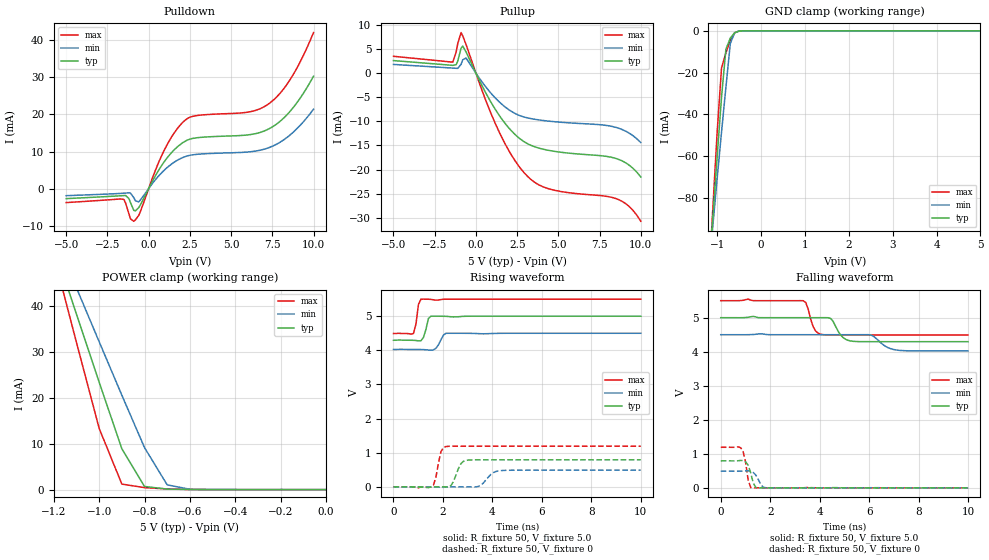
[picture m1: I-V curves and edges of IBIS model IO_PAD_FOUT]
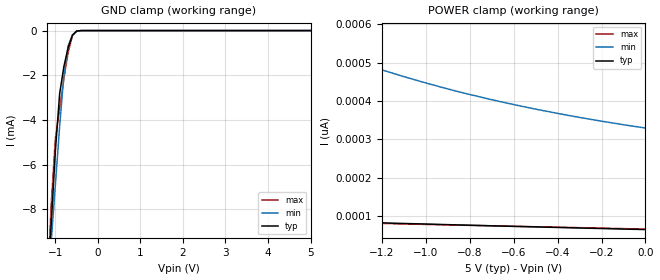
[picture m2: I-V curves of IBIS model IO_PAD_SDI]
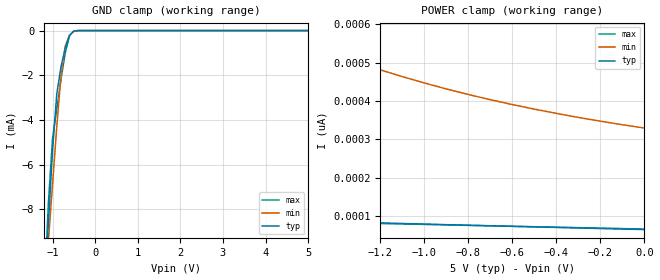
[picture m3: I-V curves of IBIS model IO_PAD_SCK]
[IBIS Ver]   3.2
[Comment Char]   |_char
[File name]   rx4111ce_5v.ibs
[File Rev]   1.0
[Date]   2019/10/04 13:08:42
[Source]
[Notes]
[Disclaimer]
This information is for modeling purposes only, and is not guaranteed.
Property of SEIKO EPSON Corp.,
unauthorized reproduction and/or distribution is strictly prohibited.
[Copyright]
Copyright 2019, SEIKO EPSON Corp.
[Component]   T5462W0A
Si_location Pin
Timing_location Pin
[Manufacturer]   SEIKO EPSON Corp.
| RX-4111CE
[Package]
R_pkg   267m   NA   NA
L_pkg   2.8nH   NA   NA
C_pkg   0.70pF   NA   NA
[Pin] signal_name   model_name
1   VDD   POWER
2   VBAT   POWER
3   DI   IO_PAD_SDI
4   FOUT   IO_PAD_FOUT
5   CLK   IO_PAD_SCK
6   DO   IO_PAD_SDO
7   CE   IO_PAD_CE
8   VIO   POWER
9   GND   GND
10   /INT   IO_PAD_XINT
| Models and submodels in the file (6): IO_PAD_FOUT (3-state), IO_PAD_SDI (Input), IO_PAD_SCK (Input), IO_PAD_SDO (3-state), IO_PAD_CE (Input), IO_PAD_XINT (Open_drain)
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[Model]   IO_PAD_FOUT
Model_type 3-state
Enable Active-High
Polarity Non-Inverting
Vmeas=2.5
C_comp   2.5p   2.0p   3.0p
[Temperature Range] 25   105   -40
[Voltage Range]   5.0   4.5   5.5
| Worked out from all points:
|   slope of the pulldown table from 0 to 0.75 V, typ, clamps not added: 126 ohm
|   slope of the pullup table from 0 to 0.75 V, typ, clamps not added: 149 ohm
|   GND clamp passes 1 mA (typ) near -0.60 V on its own axis
|   POWER clamp passes 1 mA (typ) near -0.80 V on its own axis
|   falling waveform, R_fixture 50, V_fixture 5.0: 20-80 % time 354ps typ, 503ps min, 257ps max; typ from 5 V to 4.29 V
|   falling waveform, R_fixture 50, V_fixture 0: 20-80 % time 185ps typ, 230ps min, 167ps max; typ from 0.793 V to 0 V
|   rising waveform, R_fixture 50, V_fixture 5.0: 20-80 % time 152ps typ, 215ps min, 119ps max; typ from 4.29 V to 5 V
|   rising waveform, R_fixture 50, V_fixture 0: 20-80 % time 269ps typ, 381ps min, 199ps max; typ from 0 V to 0.793 V
[Pullup]
-5V       2.598mA    1.801mA    3.488mA
-1.4V     1.602mA    1.04mA     2.29mA
-1.2V     1.734mA    995.3uA    4.356mA
-900mV    5.147mA    1.814mA    8.407mA
-600mV    4.408mA    3.126mA    5.954mA
1.2V      -7.642mA   -5.236mA   -10.62mA
2.1V      -11.76mA   -7.82mA    -16.67mA
3V        -14.38mA   -9.175mA   -20.93mA
4.5V      -16.07mA   -9.985mA   -24.05mA
8.6V      -17.81mA   -11.36mA   -26.14mA
9.4V      -19.36mA   -12.67mA   -28mA
10V       -21.52mA   -14.39mA   -30.72mA
[Pulldown]
-5V       -2.695mA   -1.899mA   -3.76mA
-1.5V     -1.871mA   -1.232mA   -2.909mA
-1.1V     -3.756mA   -1.223mA   -8.145mA
-900mV    -5.868mA   -2.416mA   -8.805mA
-600mV    -5.116mA   -3.564mA   -7.202mA
900mV     6.952mA    4.772mA    9.936mA
2V        12.16mA    8.239mA    17.55mA
2.7V      13.56mA    9.131mA    19.52mA
6.1V      14.53mA    9.907mA    20.68mA
7.3V      16.12mA    11.06mA    22.91mA
8.6V      20.95mA    14.55mA    29.52mA
10V       30.3mA     21.42mA    42.06mA
[GND Clamp]
-5V       -1.289A    -1.043A    -1.612A
-1.2V     -119.6mA   -117.1mA   -123.7mA
-1.1V     -89.89mA   -93.83mA   -85.8mA
-1V       -60.42mA   -70.86mA   -48.73mA
-900mV    -31.79mA   -48.51mA   -17.79mA
-800mV    -8.762mA   -26.99mA   -10.57mA
-700mV    -3.482mA   -6.087mA   -4.558mA
-600mV    -875.1uA   -938.3uA   -964.6uA
-500mV    -86.79uA   -136.7uA   -53.06uA
-400mV    -4.756uA   -14.79uA   -1.084uA
5V        63.88pA    6.455uA    39.96pA
[POWER Clamp]
-5V       627.4mA    509.9mA    781.1mA
-1.2V     53.06mA    55.67mA    50.97mA
-1.1V     38.19mA    43.92mA    32.03mA
-1V       23.39mA    32.21mA    13.34mA
-900mV    8.899mA    20.56mA    1.198mA
-800mV    681.2uA    9.149mA    429.9uA
-700mV    117.2uA    1.034mA    142uA
-600mV    22.79uA    76.25uA    23.1uA
0V        63.54pA    1.113nA    49.41pA
[Falling Waveform]
R_fixture=50
V_fixture=5.0
V_fixture_min=4.5
V_fixture_max=5.5
0s        5V         4.5V       5.5V
3.333ns   5V         4.5V       5.499V
3.838ns   5V         4.5V       4.608V
4.141ns   5V         4.5V       4.501V
4.444ns   4.977V     4.5V       4.493V
4.848ns   4.489V     4.5V       4.492V
5.253ns   4.316V     4.5V       4.492V
6.061ns   4.295V     4.492V     4.492V
7.172ns   4.295V     4.044V     4.492V
10ns      4.295V     4.024V     4.492V
[Falling Waveform]
R_fixture=50
V_fixture=0
V_fixture_min=0
V_fixture_max=0
0s        793.4mV    489.5mV    1.193V
808.1ps   805.6mV    490.2mV    1.178V
909.1ps   802.1mV    494.8mV    1.058V
1.01ns    763mV      499.2mV    734.5mV
1.111ns   664.1mV    500.2mV    224mV
1.212ns   439.3mV    488.6mV    10.14mV
1.414ns   12.91mV    379mV      74.07uV
1.616ns   264.6uV    106.9mV    -4.661uV
1.818ns   -9.787uV   3.8mV      -18.98uV
10ns      0V         0V         0V
[Rising Waveform]
R_fixture=50
V_fixture=5.0
V_fixture_min=4.5
V_fixture_max=5.5
0s        4.295V     4.024V     4.492V
808.1ps   4.294V     4.025V     4.493V
909.1ps   4.289V     4.024V     4.763V
1.01ns    4.277V     4.024V     5.343V
1.111ns   4.282V     4.024V     5.499V
1.212ns   4.375V     4.021V     5.5V
1.414ns   4.934V     4.01V      5.497V
1.515ns   4.999V     4.005V     5.492V
2.121ns   4.997V     4.499V     5.499V
10ns      5V         4.5V       5.5V
[Rising Waveform]
R_fixture=50
V_fixture=0
V_fixture_min=0
V_fixture_max=0
0s        0V         0V         0V
1.616ns   96.93uV    -1.137mV   51.94mV
1.919ns   -648.9uV   -11.19mV   1.033V
2.121ns   -2.477mV   -4.226mV   1.182V
2.323ns   37mV       -40.99uV   1.19V
2.727ns   680.2mV    7.872uV    1.192V
3.03ns    784.9mV    -1.033mV   1.193V
3.434ns   792.1mV    13.43mV    1.193V
4.343ns   793.3mV    476.9mV    1.193V
10ns      793.4mV    489.5mV    1.193V
[Ramp]
R_load=50
dV/dt_r   4.760E-1/2.599E-10   2.937E-1/3.667E-10   7.157E-1/1.807E-10
dV/dt_f   4.228E-1/3.439E-10   2.856E-1/5.027E-10   6.049E-1/2.422E-10
|[End   IO_PAD_FOUT
[Model]   IO_PAD_SDI
Model_type Input
Enable Active-High
Polarity Non-Inverting
Vinh=4.4
Vinl=0.9
C_comp   2.5p   2.0p   3.0p
[Temperature Range] 25   105   -40
[Voltage Range]   5.0   4.5   5.5
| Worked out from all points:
|   GND clamp passes 1 mA (typ) near -0.73 V on its own axis
[GND Clamp]
-5V       -144.1mA   -115mA     -178.6mA
-1.2V     -12.05mA   -12.06mA   -12.02mA
-1.1V     -8.699mA   -9.474mA   -7.793mA
-1V       -5.361mA   -6.879mA   -4.813mA
-900mV    -2.819mA   -4.28mA    -3.497mA
-800mV    -1.604mA   -1.983mA   -2.157mA
-700mV    -762.3uA   -688.3uA   -983.1uA
-600mV    -207.7uA   -196.5uA   -228.8uA
-500mV    -21.87uA   -34.46uA   -13.49uA
-300mV    -47nA      -340.4nA   -3.539nA
5V        64.78pA    378.7pA    60.01pA
[POWER Clamp]
-5V       175.7pA    2.756nA    8.229uA
-4.7V     164.3pA    2.408nA    4.054nA
-4.6V     161pA      2.301nA    164pA
-4.5V     157.5pA    2.198nA    120.6pA
-3V       116.1pA    1.074nA    102.1pA
-1.7V     90.46pA    588.6pA    86.56pA
-1.6V     88.84pA    564.3pA    85.39pA
-1.4V     85.46pA    520pA      82.84pA
-1.2V     82.29pA    481pA      80.5pA
-900mV    77.56pA    431.2pA    76.87pA
-500mV    71.72pA    378.6pA    72.15pA
0V        64.78pA    329.4pA    66.08pA
[Model]   IO_PAD_SCK
Model_type Input
Enable Active-High
Polarity Non-Inverting
Vinh=4.4
Vinl=0.9
C_comp   2.5p   2.0p   3.0p
[Temperature Range] 25   105   -40
[Voltage Range]   5.0   4.5   5.5
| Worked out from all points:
|   GND clamp passes 1 mA (typ) near -0.73 V on its own axis
[GND Clamp]
-5V       -144.1mA   -115mA     -178.6mA
-1.2V     -12.05mA   -12.06mA   -12.02mA
-1.1V     -8.699mA   -9.474mA   -7.793mA
-1V       -5.361mA   -6.879mA   -4.813mA
-900mV    -2.819mA   -4.28mA    -3.497mA
-800mV    -1.604mA   -1.983mA   -2.157mA
-700mV    -762.3uA   -688.3uA   -983.1uA
-600mV    -207.7uA   -196.5uA   -228.8uA
-500mV    -21.87uA   -34.46uA   -13.49uA
-300mV    -47nA      -340.4nA   -3.539nA
5V        64.77pA    378.7pA    60.03pA
[POWER Clamp]
-5V       175.7pA    2.756nA    8.229uA
-4.7V     164.3pA    2.408nA    4.054nA
-4.6V     161pA      2.301nA    164.1pA
-4.5V     157.5pA    2.198nA    120.7pA
-3V       116.1pA    1.074nA    102.1pA
-1.7V     90.45pA    588.6pA    86.59pA
-1.6V     88.83pA    564.3pA    85.41pA
-1.4V     85.45pA    520pA      82.87pA
-1.2V     82.28pA    480.9pA    80.52pA
-900mV    77.55pA    431.2pA    76.89pA
-500mV    71.71pA    378.6pA    72.17pA
0V        64.78pA    329.4pA    66.1pA
